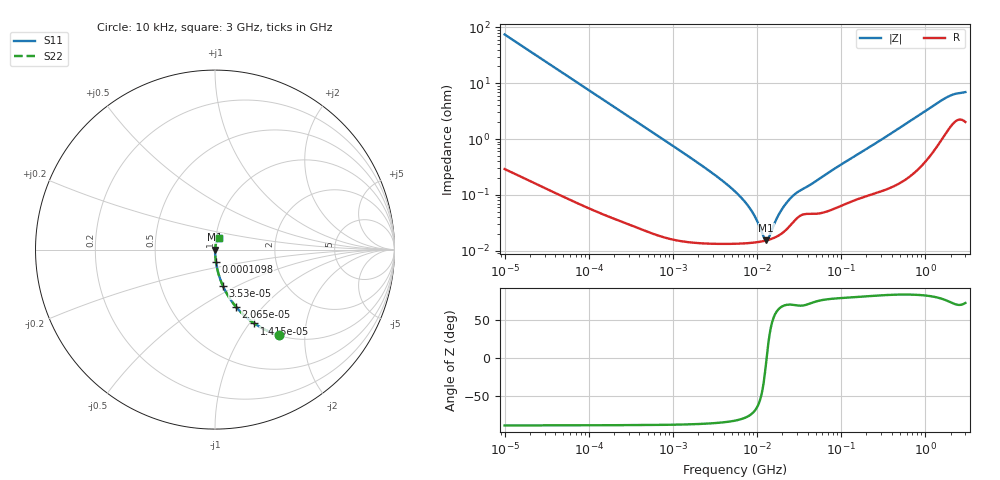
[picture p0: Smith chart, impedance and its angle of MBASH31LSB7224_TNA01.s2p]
! MBASH31LSB7224_TNA01  S-PARAMETER MODEL  ( Standard Model )
! Model Generated by TAIYO YUDEN Corporation (http://www.ty-top.com)
! Version 1.0
! TAIYO YUDEN Control No. 220601
! Copyright(c) 2013 TAIYO YUDEN CO.,LTD. All Rights Reserved.
! Product Description (link to TY-COMPAS)
! https://ds.yuden.co.jp/TYCOMPAS/or/detail?pn=MBASH31LSB7224KTNA01&u=M
! Products Name : Multilayer Ceramic Capacitors
! Characteristics :
!  Capacitance : 0.22 [uF] , Rated Voltage : 100 [V] , TCC : X7R
!  Case Size : 3.2 x 1.6 / 0.126 x 0.063 [mm/inch] , Thickness : 1.6 / 0.063 [mm/inch]
!  (Conditions: Temperature = 25 [degC] , DC Bias Voltage = 0 [V])
! External Node Assignments :
!  1  o---| |---o  2
! GND o---------o GND
! Frequency Range : 10kHz  -  3GHz  [ 401 STEP ]
# MHZ S RI R 50
! Freq[MHz].  S11 Real  S11 Imag  S21 Real  S21 Imag  S12 Real  S12 Imag  S22 Real  S22 Imag
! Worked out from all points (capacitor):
!   401 points, 10 kHz to 3 GHz, reference 50 ohm
!   read as one part in series: C = 213 nF near 10.65 kHz
!   lowest |Z| = 15.3 mohm at 12.83 MHz (marker M1)
!   series resonance near 13.02 MHz, so ESL is about 700 pH
!   S11 on the Smith chart (normalised r, x): 10 kHz: 1.01, -1.49; 14.15 kHz: 1.00, -1.06; 20.65 kHz: 1.00, -0.72; 35.3 kHz: 1.00, -0.42; 109.8 kHz: 1.00, -0.14; 3 GHz: 1.04, +0.13
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0.01  0.3586 -0.4777  0.6414 0.4777  0.6414 0.4777  0.3586 -0.4777
0.014146  0.2193 -0.4116  0.7807 0.4116  0.7807 0.4116  0.2193 -0.4116
0.020651  0.1172 -0.3193  0.8828 0.3193  0.8828 0.3193  0.1172 -0.3193
0.035295  0.0442 -0.2027  0.9558 0.2027  0.9558 0.2027  0.0442 -0.2027
0.082683  0.00883 -0.0901  0.9912 0.0901  0.9912 0.0901  0.00883 -0.0901
0.109813  0.00521 -0.0681  0.9948 0.0681  0.9948 0.0681  0.00521 -0.0681
0.683653  0.000307 -0.0111  0.9997 0.0111  0.9997 0.0111  0.000307 -0.0111
2.737278  0.000141 -0.00266  0.9999 0.00266  0.9999 0.00266  0.000141 -0.00266
5.477226  0.000134 -0.00115  0.9999 0.00115  0.9999 0.00115  0.000134 -0.00115
8.516475  0.000138 -0.000514  0.9999 0.000514  0.9999 0.000514  0.000138 -0.000514
9.97066  0.000142 -0.000318  0.9999 0.000318  0.9999 0.000318  0.000142 -0.000318
12.04705  0.000149 -9.19e-05  0.9999 9.19e-05  0.9999 9.19e-05  0.000149 -9.19e-05
12.83117  0.000152 -1.73e-05  0.9998 1.73e-05  0.9998 1.73e-05  0.000152 -1.73e-05
14.10408  0.000158 9.48e-05  0.9998 -9.48e-05  0.9998 -9.48e-05  0.000158 9.48e-05
18.73182  0.000193 0.000443  0.9998 -0.000443  0.9998 -0.000443  0.000193 0.000443
23.35767  0.000256 0.000732  0.9997 -0.000732  0.9997 -0.000732  0.000256 0.000732
30.05882  0.000385 0.00104  0.9996 -0.00104  0.9996 -0.00104  0.000385 0.00104
45.28751  0.000458 0.00152  0.9995 -0.00152  0.9995 -0.00152  0.000458 0.00152
374.4521  0.00146 0.0119  0.9985 -0.0119  0.9985 -0.0119  0.00146 0.0119
1700.79  0.0142 0.0506  0.9858 -0.0506  0.9858 -0.0506  0.0142 0.0506
2188.735  0.0226 0.0579  0.9774 -0.0579  0.9774 -0.0579  0.0226 0.0579
3000  0.024 0.0635  0.976 -0.0635  0.976 -0.0635  0.024 0.0635
